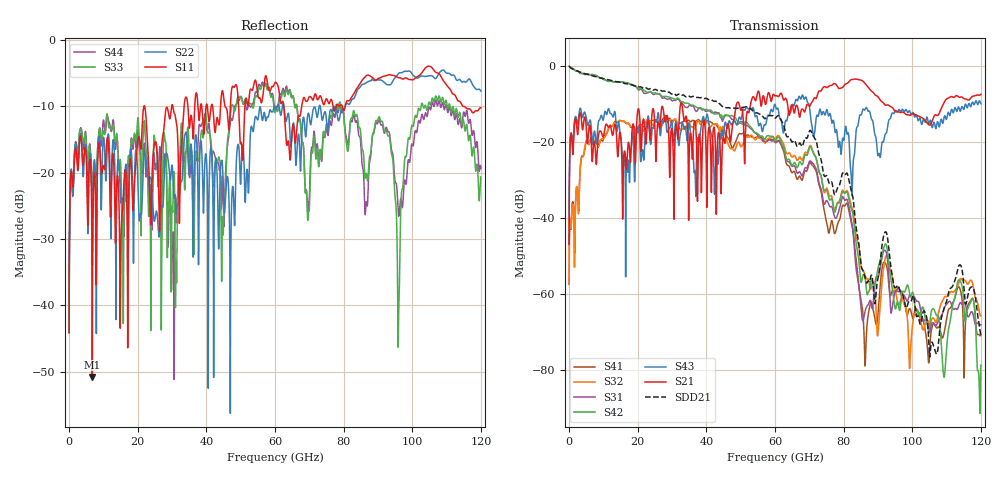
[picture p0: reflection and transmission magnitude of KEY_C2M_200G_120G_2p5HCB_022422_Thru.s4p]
! Touchstone file
!  Generated:  9:04:18 AM  Nov 09, 2021
!  Setup:  LinearFrequency
!  Solution:  LinearFrequency
# GHz S MA R 50.000000
! Terminal data exported
! Port[1] = P1
! Port[2] = P3
! Port[3] = P2
! Port[4] = P4
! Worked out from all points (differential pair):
!   12000 points, 10 MHz to 120 GHz, reference 50 ohm
!   strongest paths, dB at 10 MHz, 30.01 GHz, 60.01 GHz, 90.01 GHz, 120 GHz:
!     S21: -47.0, -16.9, -7.9, -8.1, -7.5
!     S43: -47.0, -15.0, -10.1, -23.6, -9.9
!     S42: -0.1, -8.5, -19.8, -53.3, -78.7
!     S31: -0.1, -9.2, -19.9, -55.4, -68.1
!     S32: -57.5, -15.1, -19.2, -70.4, -65.8
!     S41: -57.5, -14.5, -20.1, -65.5, -70.8
!   taken as a pair (ports 2,1 in; 4,3 out), SDD21 dB: -0.1, -7.4, -13.7, -55.9, -71.0
!   lowest |S11| = -50.8 dB at 6.77 GHz (marker M1), VSWR 1.01, Z = 49.9 - j0.262 ohm
!   |S11| at or under -10 dB: start of sweep to 21.81 GHz; 22.03 GHz to 29.89 GHz (7.857 GHz wide, 30.3 % of centre); 114.8 GHz to end of sweep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
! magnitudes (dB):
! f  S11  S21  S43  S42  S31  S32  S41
! 10 MHz  -44.1  -47.0  -47.0  -0.1  -0.1  -57.5  -57.5
! 6.77 GHz  -50.8  -25.2  -20.3  -2.3  -2.2  -19.0  -19.1
! 61.07 GHz  -7.3  -8.0  -12.1  -18.8  -19.6  -18.4  -19.7
! 81.13 GHz  -9.1  -4.6  -17.9  -33.5  -35.4  -33.0  -36.4
! 86.31 GHz  -5.5  -4.7  -11.4  -56.1  -64.3  -55.2  -78.6
! 91.93 GHz  -5.4  -10.2  -18.6  -47.2  -48.5  -51.6  -51.7
! 120 GHz  -10.2  -7.5  -9.9  -78.7  -68.1  -65.8  -70.8
